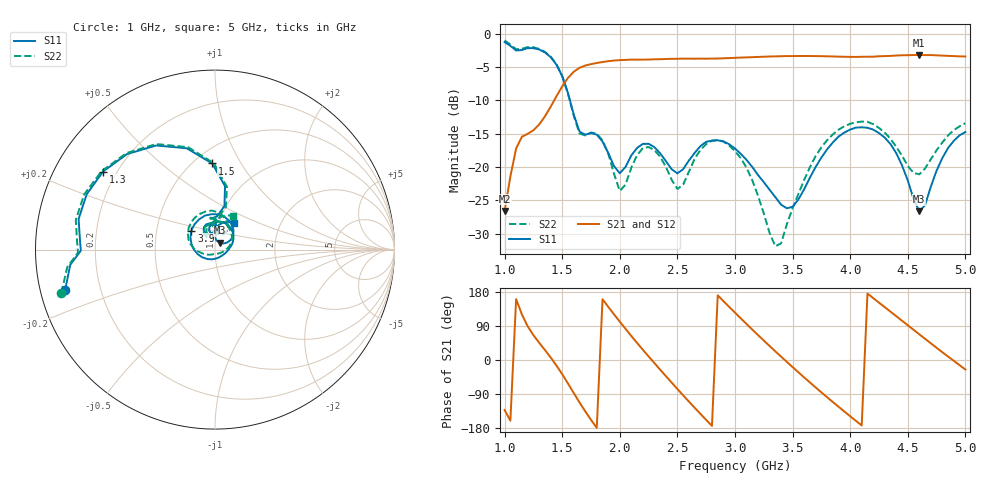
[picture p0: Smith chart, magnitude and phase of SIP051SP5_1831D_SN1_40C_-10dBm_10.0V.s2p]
# GHz  S  dB  R  50
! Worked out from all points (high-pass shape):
!   81 points, 1 GHz to 5 GHz, reference 50 ohm
!   highest |S21| = -3.19 dB at 4.6 GHz (marker M1); lowest = -26.6 dB at 1 GHz (marker M2)
!   |S21| within 3 dB of the highest: 1.575 GHz to end of sweep
!   lowest |S11| = -26.7 dB at 4.6 GHz (marker M3), VSWR 1.10, Z = 52.5 + j4.07 ohm
!   |S11| at or under -10 dB: 1.567 GHz to end of sweep
!   |S22| runs from -31.9 to -1.0 dB; largest |S21 - S12| = 0.003
!   S11 on the Smith chart (normalised r, x): 1 GHz: 0.07, -0.13; 1.3 GHz: 0.15, +0.31; 1.5 GHz: 0.61, +0.76; 3.9 GHz: 0.75, +0.16; 5 GHz: 1.17, +0.36
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1  -1.26 -164.9  -26.62 -131.9  -26.57 -131.8  -1.02 -164.3
1.1  -2.53 -179.6  -17.23 160.7  -17.22 160.9  -2.34 -178.8
1.3  -2.38 145.1  -13.63 45.6  -13.64 45.6  -2.29 145.4
1.5  -6.37 91.9  -7.91 -37.4  -7.90 -37.4  -6.35 90.7
1.6  -12.10 77.8  -5.72 -87.0  -5.71 -87.1  -12.31 75.7
1.7  -15.16 96.5  -4.78 -135.4  -4.79 -135.4  -15.27 98.0
1.85  -16.18 88.8  -4.25 160.3  -4.25 160.3  -16.02 84.4
2  -20.95 105.8  -3.97 101.0  -3.97 101.0  -23.60 100.1
2.2  -16.54 109.5  -3.89 27.1  -3.90 27.1  -17.17 114.4
2.35  -17.94 88.7  -3.83 -25.4  -3.83 -25.4  -18.46 88.7
2.6  -19.03 107.1  -3.75 -109.8  -3.75 -109.8  -20.71 116.7
2.8  -16.06 80.7  -3.74 -173.8  -3.74 -173.9  -16.06 90.7
3  -17.23 43.5  -3.63 125.0  -3.61 125.0  -17.62 46.7
3.2  -21.21 9.9  -3.49 65.8  -3.50 65.8  -24.33 -1.1
3.4  -25.66 -37.8  -3.38 8.9  -3.38 8.9  -31.47 -108.2
3.7  -20.00 -165.6  -3.37 -72.4  -3.38 -72.4  -18.36 176.0
3.9  -15.43 141.2  -3.45 -123.5  -3.45 -123.8  -14.40 140.1
4.1  -14.05 95.4  -3.47 -172.7  -3.47 -172.7  -13.19 102.9
4.35  -16.56 45.9  -3.34 127.5  -3.33 127.5  -15.78 64.5
4.6  -26.68 56.6  -3.19 67.8  -3.20 67.7  -21.10 78.0
4.8  -18.65 88.1  -3.30 20.5  -3.29 20.7  -16.32 91.3
5  -14.76 55.5  -3.42 -25.0  -3.43 -24.9  -13.43 62.5
